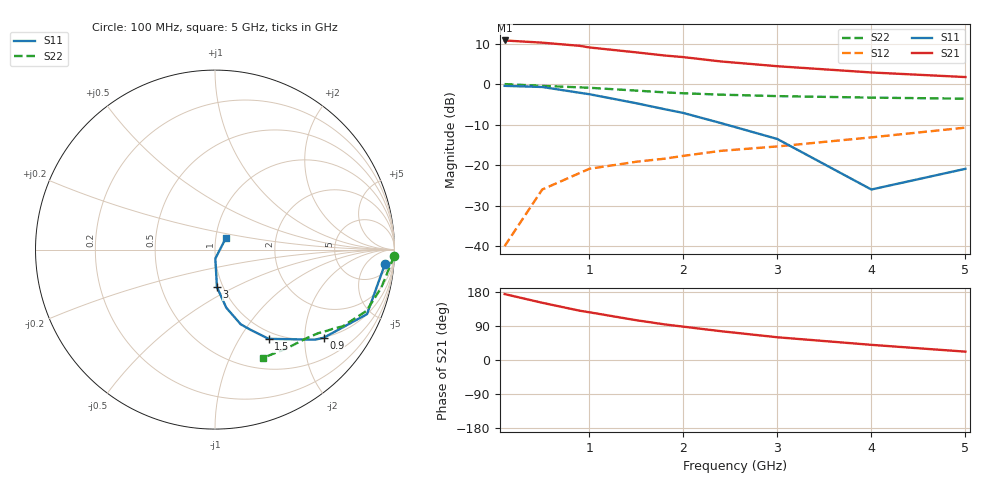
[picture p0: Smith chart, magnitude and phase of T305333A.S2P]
!AT-30533
!S and NOISE PARAMETERS at Vce=2.7V  Ic=1mA.  LAST UPDATED 06-23-94
# ghz s ma r 50!
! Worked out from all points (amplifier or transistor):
!   11 points, 100 MHz to 5 GHz, reference 50 ohm
!   highest |S21| = 10.8 dB at 100 MHz (marker M1)
!   |S21| within 3 dB of that: start of sweep to 1.524 GHz
!   unconditionally stable (mu >= 1): 2.694 GHz to 4.571 GHz
!   at 500 MHz: K = 0.26, MSG = 18.1 dB, |S12| = -26.0 dB
!   at 1.8 GHz: K = 0.82, MSG = 12.7 dB, |S12| = -18.4 dB
!   at 5 GHz: K = 0.97, MSG = 6.2 dB, |S12| = -10.8 dB
!   lowest NFmin = 0.30 dB at 500 MHz
!   S11 on the Smith chart (normalised r, x): 100 MHz: 10, -17; 900 MHz: 0.99, -2.48; 1.5 GHz: 0.90, -1.35; 3 GHz: 0.94, -0.41; 5 GHz: 1.12, +0.15
0.1  0.95 -5.0  3.45 174.0  0.01 87.0  0.999 -2.0
0.5  0.92 -23.0  3.24 151.0  0.05 74.0  0.95 -13.0
0.9  0.78 -39.0  2.96 130.0  0.08 64.0  0.91 -22.0
1  0.75 -42.0  2.83 126.0  0.09 63.0  0.9 -23.0
1.5  0.58 -59.0  2.46 105.0  0.11 55.0  0.83 -31.0
1.8  0.49 -66.0  2.25 94.0  0.12 53.0  0.79 -34.0
2  0.44 -71.0  2.15 88.0  0.13 52.0  0.77 -36.0
2.4  0.33 -79.0  1.9 76.0  0.15 51.0  0.74 -39.0
3  0.21 -87.0  1.66 60.0  0.17 51.0  0.71 -44.0
4  0.05 -88.0  1.39 40.0  0.22 52.0  0.68 -54.0
5  0.09 47.0  1.22 22.0  0.29 49.0  0.66 -66.0
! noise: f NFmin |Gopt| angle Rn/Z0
0.5  0.3  0.94  7  1.02
0.9  0.4  0.89  16  0.88
1.8  0.9  0.75  43  0.58
2.4  1.3  0.65  65  0.38
